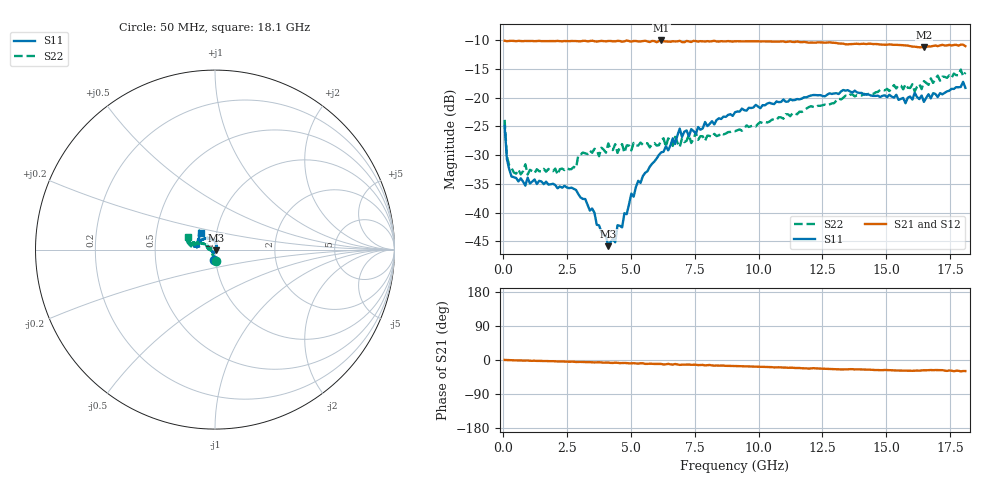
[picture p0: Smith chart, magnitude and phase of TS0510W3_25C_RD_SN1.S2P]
! Network Analyzer HP8720D.06.14 Serial No. US36140669
! 17 Jun 2005  07:51:15
! Frequency  S11  S21  S12  S22
# HZ  S  DB R 50
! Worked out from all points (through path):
!   201 points, 50 MHz to 18.1 GHz, reference 50 ohm
!   highest |S21| = -10.04 dB at 6.187 GHz (marker M1); lowest = -11.2 dB at 16.48 GHz (marker M2)
!   group delay of S21, straight-line fit = 4.79 ps
!   lowest |S11| = -45.8 dB at 4.111 GHz (marker M3), VSWR 1.01, Z = 50.4 - j0.317 ohm
!   |S11| at or under -10 dB: start of sweep to end of sweep
!   |S22| runs from -33.4 to -15.1 dB; largest |S21 - S12| = 0.0094
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5e7  -24.89 -95.1  -10.10 0.1  -10.12 0.1  -23.86 -82.8
1.4025e8  -30.69 -108.8  -10.17 -0.2  -10.16 -0.2  -30.22 -118.9
5.0125e8  -33.97 -132.5  -10.17 -1.0  -10.15 -1.0  -33.22 -159.6
8.6225e8  -35.30 -140.3  -10.13 -1.4  -10.17 -1.3  -31.58 -168.8
9.525e8  -33.90 -136.7  -10.15 -1.3  -10.15 -1.6  -33.37 -172.0
2.12575e9  -35.76 -116.0  -10.12 -3.8  -10.16 -3.7  -33.37 165.8
2.84775e9  -36.05 -93.9  -10.15 -5.3  -10.17 -5.0  -32.23 156.8
3.1185e9  -37.61 -108.3  -10.11 -5.3  -10.17 -5.4  -29.53 175.4
3.75025e9  -42.21 -77.4  -10.18 -5.9  -10.22 -5.9  -30.18 172.6
4.11125e9  -45.83 -38.0  -10.14 -6.8  -10.13 -7.1  -27.95 171.5
4.65275e9  -42.56 28.4  -10.26 -8.0  -10.17 -7.9  -28.07 175.6
5.2845e9  -34.46 62.2  -10.22 -9.6  -10.19 -9.8  -28.32 163.3
6.09675e9  -29.95 75.5  -10.15 -10.1  -10.09 -10.2  -28.25 165.9
6.187e9  -29.50 84.1  -10.04 -10.3  -10.13 -10.6  -27.38 159.0
6.7285e9  -28.06 88.0  -10.21 -10.6  -10.29 -11.2  -26.81 160.7
6.909e9  -25.38 90.1  -10.10 -12.9  -10.20 -12.5  -28.59 155.8
7.27e9  -26.74 88.0  -10.23 -12.0  -10.25 -12.7  -26.45 158.4
9.075e9  -22.54 120.2  -10.19 -15.9  -10.19 -15.9  -25.83 150.4
1.21435e10  -19.54 163.8  -10.42 -21.6  -10.41 -21.7  -21.60 155.0
1.512175e10  -19.50 169.6  -10.73 -26.8  -10.71 -26.4  -18.85 165.6
1.64755e10  -20.73 160.5  -11.25 -27.0  -11.19 -26.4  -17.11 164.6
1.81e10  -18.28 130.9  -11.03 -29.2  -11.02 -30.7  -15.62 155.5
